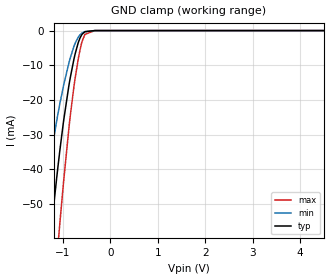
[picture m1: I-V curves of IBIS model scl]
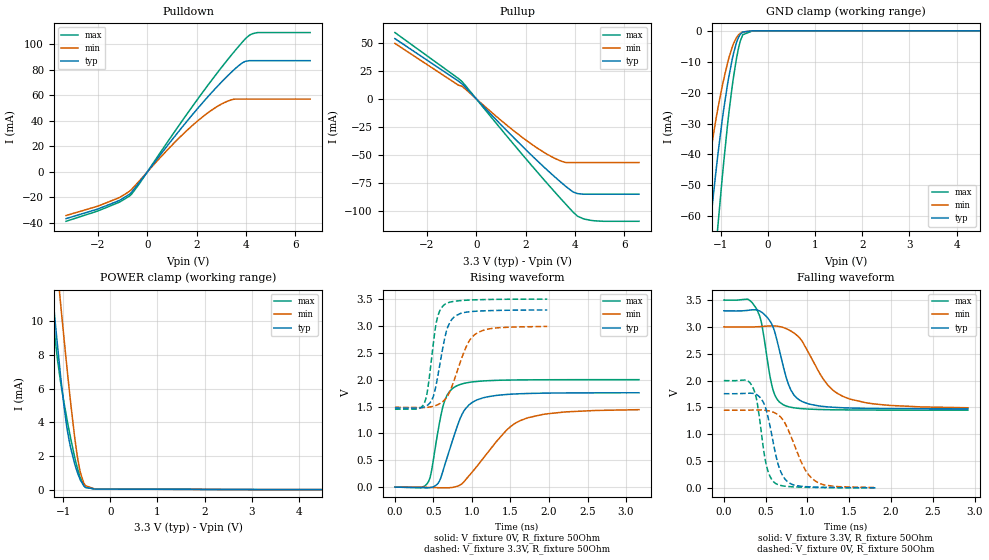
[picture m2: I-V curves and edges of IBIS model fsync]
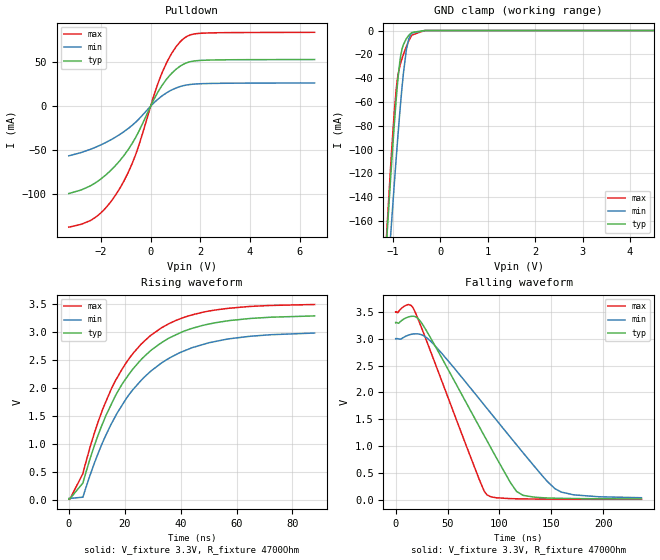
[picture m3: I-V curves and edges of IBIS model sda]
|Texas Instruments Incorporated
|50-W, 2-MHz Digital Input 4-Channel Automotive Class-D Audio Amplifier
|With Load Dump Protection and I2C Diagnostics
|Marketing part#   Digital Voltage Range   Package-type   #pins
|TPA6404   3V - 26.4V   HSSOP   56
[IBIS Ver]   4.1
[File name]   tpa6404-q1.ibs
[File Rev]   1.0
[Date]   10/27/2017
[Source]
| Texas Instruments Incorporated.
| Analog-eLab Design Center
| 12500 TI Blvd
| Dallas, TX -75243
[Notes]   Revision History:
| Rev 1.0: 9/17/2016
| - Initial version of the model
| - Model generated from simulations in SPECTRE
| - Model matched to SPICE simulation
| - C_comp although listed in numerical order of value are
|   obtained from varying PVT conditions. For PVT conditions for
|   each specific value refer the buffer description under
|   respective [Model]. IBIS model user is responsible for using
|   appropriate C_comp to simulate for Signal Integrity.
[Disclaimer]
| This model is designed as an aid for customers of Texas Instruments.
| TI and its licensors and suppliers make no warranties, either expressed
| or implied, with respect to this  model, including the warranties of
| merchantability or fitness for a particular purpose. The model is
| provided solely on an "as is" basis. The entire risk as to its quality
| and performance is with the customer.
[Copyright]
(C) Copyright 2017 Texas Instruments Incorporated.All rights reserved.
|   TPA6404_Q1DKQ
[Component]   TPA6404QDKQQ1
[Manufacturer]   TI
[Package]   |56 DKQ - HSSOP Package
|   typ   min   max
R_pkg   0.2   0.16   0.24
L_pkg   1.5nH   1.2nH   1.8nH
C_pkg   0.4pF   0.32pF   0.48pF
[Pin]  signal_name   model_name   R_pin   L_pin   C_pin
1   GND   gnd   NA   NA   NA
2   PVDD   power   NA   NA   NA
3   VBAT   power   NA   NA   NA
4   AVSS   power   NA   NA   NA
5   AVDD   power   NA   NA   NA
6   GVDD   power   NA   NA   NA
7   GVDD   power   NA   NA   NA
8   GND   gnd   NA   NA   NA
9   IN_4P   nc   NA   NA   NA
10   IN_4M   nc   NA   NA   NA
11   IN_3P   nc   NA   NA   NA
12   IN_3M   nc   NA   NA   NA
13   IN_2P   nc   NA   NA   NA
14   IN_2M   nc   NA   NA   NA
15   IN_1P   nc   NA   NA   NA
16   IN_1M   nc   NA   NA   NA
17   DVSS   gnd   NA   NA   NA
18   DVDD   power   NA   NA   NA
19   SYNC   nc   NA   NA   NA
20   SCL   scl   NA   NA   NA
21   SDA   sda   NA   NA   NA
22   I2C_ADDR0   fsync   NA   NA   NA
23   I2C_ADDR1   fsync   NA   NA   NA
24   _STANDBY   nc   NA   NA   NA
25   _MUTE   nc   NA   NA   NA
26   _FAULT   nc   NA   NA   NA
27   _WARN   nc   NA   NA   NA
28   GND   nc   NA   NA   NA
29   PVDD   power   NA   NA   NA
30   PVDD   power   NA   NA   NA
31   BST_1M   power   NA   NA   NA
32   OUT_1M   nc   NA   NA   NA
33   GND   gnd   NA   NA   NA
34   OUT_1P   nc   NA   NA   NA
35   BST_1P   power   NA   NA   NA
36   GND   gnd   NA   NA   NA
37   BST_2M   power   NA   NA   NA
38   OUT_2M   nc   NA   NA   NA
39   GND   gnd   NA   NA   NA
40   OUT_2P   nc   NA   NA   NA
41   BST_2P   power   NA   NA   NA
42   PVDD   power   NA   NA   NA
43   PVDD   power   NA   NA   NA
44   BST_3M   power   NA   NA   NA
45   OUT_3M   nc   NA   NA   NA
46   GND   gnd   NA   NA   NA
47   OUT_3P   nc   NA   NA   NA
48   BST_3P   power   NA   NA   NA
49   GND   gnd   NA   NA   NA
50   BST_4M   power   NA   NA   NA
51   OUT_4M   nc   NA   NA   NA
52   GND   gnd   NA   NA   NA
53   OUT_4P   nc   NA   NA   NA
54   BST_4P   power   NA   NA   NA
55   PVDD   power   NA   NA   NA
56   PVDD   power   NA   NA   NA
57   ThermalPad   gnd   NA   NA   NA
| Models and submodels in the file (3): scl (Input), fsync (I/O), sda (I/O_open_drain)
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|   sclk Model
[Model]   scl
Model_type   Input
Vinl = 0.99
Vinh = 2.31
|   typ   min   max
|   (nom PVT)   (fast PVT)   (slow PVT)
C_comp   6.288e-13   4.758e-13   7.537e-13
| Where nom  PVT is Nominal Process, 3.3V, 27C
|   Fast PVT is Strong Process,  3.5V, -40C
|   Slow PVT is Weak Process,   3V, 150C
[Model spec]
|subparameter
Vinl   0.99   0.90   1.05
Vinh   2.31   2.10   2.45
[Voltage Range]   3.3   3   3.5
|Junction Temperature
[Temperature Range]   27   150   -40
[Power Clamp Reference]   3.3   3   3.5
[GND Clamp Reference]   0   0   0
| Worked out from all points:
|   GND clamp passes 1 mA (typ) near -0.59 V on its own axis
[GND Clamp]
|   Voltage   I(typ)   I(min)   I(max)
-3.3V     -394.6mA   -304mA     -465.7mA
-1.544V   -99.89mA   -64.75mA   -138.1mA
-1.449V   -85.57mA   -54.72mA   -120.8mA
-1.287V   -62.45mA   -39.03mA   -92.13mA
-1.238V   -55.77mA   -34.62mA   -83.61mA
-1.105V   -39.09mA   -23.91mA   -61.71mA
-1.067V   -34.61mA   -21.1mA    -55.6mA
-877.8mV  -16.02mA   -9.452mA   -28.4mA
-769.5mV  -8.242mA   -4.556mA   -16.14mA
-642mV    -2.16mA    -1.238mA   -5.635mA
-538.5mV  -329.1uA   -291.4uA   -1.101mA
6.6V      0A         0A         0A
[POWER Clamp]
|   Voltage   I(typ)   I(min)   I(max)
-3.3V     0A         0A         0A
0V        0A         0A         0A
6.6V      0A         0A         0A
|   fsync Model
[Model]   fsync
Model_type   I/O
Polarity   Non-Inverting
Enable   Active-High
Vinl = 0.99
Vinh = 2.31
Vmeas = 1.65
Vref = 0
Cref = 2pF
Rref = 70
|   typ   min   max
|   (nom PVT)   (fast PVT)   (slow PVT)
C_comp   9.736e-13   8.094e-13   1.100e-12
| Where nom  PVT is Nominal Process, 3.3V, 27C
|   Fast PVT is Strong Process,  3.5V, -40C
|   Slow PVT is Weak Process,   3V, 150C
[Model spec]
|subparameter
Vinl   0.99   0.90   1.05
Vinh   2.31   2.10   2.45
[Voltage Range]   3.3   3   3.5
|Junction Temperature
[Temperature Range]   27   150   -40
[Pullup Reference]   3.3   3   3.5
[Pulldown Reference]   0   0   0
[Power Clamp Reference]   3.3   3   3.5
[GND Clamp Reference]   0   0   0
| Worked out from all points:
|   slope of the pulldown table from 0 to 0.495 V, typ, clamps not added: 39.4 ohm
|   slope of the pullup table from 0 to 0.495 V, typ, clamps not added: 43.1 ohm
|   GND clamp passes 1 mA (typ) near -0.58 V on its own axis
|   POWER clamp passes 1 mA (typ) near -0.70 V on its own axis
|   falling waveform, V_fixture 3.3V, R_fixture 50Ohm: 20-80 % time 195ps typ, 378ps min, 135ps max; typ from 3.3 V to 1.47 V
|   rising waveform, V_fixture 0V, R_fixture 50Ohm: 20-80 % time 257ps typ, 519ps min, 157ps max; typ from 0 V to 1.76 V
|   rising waveform, V_fixture 3.3V, R_fixture 50Ohm: 20-80 % time 149ps typ, 236ps min, 112ps max; typ from 1.47 V to 3.3 V
|   falling waveform, V_fixture 0V, R_fixture 50Ohm: 20-80 % time 154ps typ, 245ps min, 115ps max; typ from 1.76 V to 0.004 V
[Pulldown]
|   Voltage   I(typ)   I(min)   I(max)
-3.3V     -36.59mA   -34.16mA   -38.69mA
-2.079V   -29.49mA   -27.22mA   -31.04mA
-1.203V   -22.91mA   -20.65mA   -24.25mA
-647mV    -16.03mA   -13.82mA   -17.58mA
994.5mV   25.05mA    20.91mA    28.46mA
2.373V    57.15mA    45.17mA    65.81mA
2.988V    70.06mA    53mA       81.42mA
3.408V    78.14mA    56.54mA    91.58mA
3.849V    85.46mA    57.07mA    101.7mA
4.143V    87.2mA     57.07mA    107.1mA
4.481V    87.2mA     57.07mA    109.2mA
6.6V      87.2mA     57.07mA    109.2mA
[GND Clamp]
|   Voltage   I(typ)   I(min)   I(max)
-3.3V     -440mA     -341.7mA   -519.1mA
-1.534V   -111.5mA   -73.85mA   -152.9mA
-1.431V   -94.25mA   -61.6mA    -132.1mA
-1.227V   -62.33mA   -39.69mA   -92.37mA
-1.062V   -39.41mA   -24.68mA   -62.25mA
-975mV    -28.86mA   -17.95mA   -47.56mA
-867.9mV  -17.84mA   -10.78mA   -31.2mA
-762.5mV  -9.177mA   -5.256mA   -17.88mA
-633mV    -2.229mA   -1.378mA   -5.882mA
-538.5mV  -388.1uA   -364.3uA   -1.272mA
-330mV    -4.25uA    -9.019uA   -5.089uA
6.6V      0A         0A         0A
[Pullup]
|   Voltage   I(typ)   I(min)   I(max)
-3.3V     53.6mA     49.34mA    59.01mA
-724mV    15.74mA    12.1mA     18.05mA
-588mV    13.44mA    11.21mA    15.53mA
1.284V    -29.46mA   -24.34mA   -34.44mA
2.553V    -56.88mA   -45.07mA   -67.28mA
2.973V    -65.43mA   -50.65mA   -77.83mA
3.51V     -75.83mA   -56.07mA   -91.03mA
3.901V    -82.68mA   -56.8mA    -100.4mA
4.095V    -84.42mA   -56.8mA    -104.4mA
4.353V    -85.03mA   -56.8mA    -107mA
4.795V    -85.03mA   -56.8mA    -108.7mA
6.6V      -85.03mA   -56.8mA    -109.2mA
[POWER Clamp]
|   Voltage   I(typ)   I(min)   I(max)
-3.3V     78.62mA    81.34mA    82.98mA
-1.294V   13.67mA    18.15mA    12.46mA
-1.224V   11.54mA    16.02mA    10.33mA
-1.123V   8.586mA    13.02mA    7.731mA
-1.056V   6.746mA    11.05mA    6.397mA
-976.8mV  4.8mA      8.789mA    5.06mA
-871mV    2.867mA    5.898mA    3.45mA
-696mV    993.8uA    1.895mA    1.238mA
-636.5mV  569.5uA    1.011mA    691.4uA
-525mV    128.3uA    227.9uA    131.5uA
-264mV    32.56uA    34.05uA    33.82uA
6.6V      0A         0A         0A
[Ramp]
R_load = 50
|   typ   min   max
dV/dt_r   1.05398/2.56961e-10   0.869396/5.22864e-10   1.20008/1.57028e-10
dV/dt_f   1.09538/1.94389e-10   0.908068/3.80996e-10   1.2297/1.34491e-10
[Falling Waveform]
V_fixture = 3.3V
V_fixture_min = 3V
V_fixture_max = 3.5V
R_fixture = 50Ohm
|   Time   V(typ)   V(min)   V(max)
0s        3.3V       3V         3.5V
281.6ps   3.308V     2.998V     3.519V
382.7ps   3.32V      3.002V     3.358V
452.5ps   3.275V     3.009V     3.06V
590ps     2.996V     3.02V      1.822V
729.9ps   2.15V      2.979V     1.537V
909.1ps   1.634V     2.791V     1.481V
1.197ns   1.517V     2.013V     1.46V
1.428ns   1.494V     1.704V     1.455V
2.92ns    1.474V     1.494V     1.45V
[Rising Waveform]
V_fixture = 0V
V_fixture_min = 0V
V_fixture_max = 0V
R_fixture = 50Ohm
|   Time   V(typ)   V(min)   V(max)
0s        345.2pV    23.28nV    146.2pV
432.7ps   -12.69mV   -4.635mV   96.19mV
471.2ps   -5.458mV   -6.65mV    271.6mV
564.5ps   79.77mV    -11.33mV   1.087V
644.3ps   400.1mV    -13.85mV   1.602V
816.8ps   1.164V     20.23mV    1.894V
919.8ps   1.465V     140.5mV    1.938V
1.062ns   1.621V     383.8mV    1.966V
1.635ns   1.738V     1.242V     1.995V
3.168ns   1.756V     1.441V     2V
[Rising Waveform]
V_fixture = 3.3V
V_fixture_min = 3V
V_fixture_max = 3.5V
R_fixture = 50Ohm
|   Time   V(typ)   V(min)   V(max)
0s        1.474V     1.486V     1.45V
382.7ps   1.495V     1.481V     1.569V
429ps     1.531V     1.487V     1.856V
496.4ps   1.679V     1.504V     2.646V
540ps     1.94V      1.524V     3.083V
647.9ps   2.784V     1.629V     3.401V
771.7ps   3.171V     2.003V     3.458V
911.6ps   3.253V     2.567V     3.477V
1.039ns   3.272V     2.841V     3.485V
1.977ns   3.297V     2.991V     3.498V
[Falling Waveform]
V_fixture = 0V
V_fixture_min = 0V
V_fixture_max = 0V
R_fixture = 50Ohm
|   Time   V(typ)   V(min)   V(max)
0s        1.757V     1.449V     2V
346ps     1.763V     1.452V     1.876V
399.8ps   1.733V     1.454V     1.584V
510ps     1.438V     1.445V     416.5mV
616.5ps   649mV      1.394V     86.83mV
681.2ps   303.6mV    1.319V     46.63mV
765.1ps   113mV      1.1V       27.92mV
972.2ps   25.29mV    342mV      13.23mV
1.087ns   16.68mV    137mV      9.613mV
1.817ns   3.697mV    8.046mV    2.24mV
|   sda Model
[Model]   sda
Model_type   I/O_open_drain
Polarity   Non-Inverting
Vinl = 0.99
Vinh = 2.31
Vmeas = 1.65
Vref = 3.3
Cref = 2pF
Rref = 4700
|   typ   min   max
|   (nom PVT)   (fast PVT)   (slow PVT)
C_comp   1.956e-12   1.803e-12   2.012e-12
| Where nom  PVT is Nominal Process, 3.3V, 27C
|   Fast PVT is Strong Process,  3.5V, -40C
|   Slow PVT is Weak Process,   3V, 150C
[Model spec]
|subparameter
Vinl   0.99   0.90   1.05
Vinh   2.31   2.10   2.45
[Voltage Range]   3.3   3   3.5
|Junction Temperature
[Temperature Range]   27   150   -40
[Pullup Reference]   3.3   3   3.5
[Pulldown Reference]   0   0   0
[Power Clamp Reference]   3.3   3   3.5
[GND Clamp Reference]   0   0   0
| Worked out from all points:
|   slope of the pulldown table from 0 to 0.495 V, typ, clamps not added: 19.9 ohm
|   falling waveform, V_fixture 3.3V, R_fixture 4700Ohm: 20-80 % time 55.9ns typ, 75ns min, 41.1ns max; typ from 3.3 V to 0.016 V
|   rising waveform, V_fixture 3.3V, R_fixture 4700Ohm: 20-80 % time 21.3ns typ, 22.8ns min, 19.9ns max; typ from 0.012 V to 3.29 V
[Pulldown]
|   Voltage   I(typ)   I(min)   I(max)
-3.3V     -99.17mA   -56.36mA   -137.3mA
-2.187V   -86.26mA   -46.17mA   -125.4mA
-1.653V   -74.09mA   -38.9mA    -110.1mA
-1.267V   -62.56mA   -32.47mA   -94.28mA
-914.1mV  -49.53mA   -25.48mA   -75.62mA
-615mV    -35.89mA   -18.39mA   -55.51mA
141mV     8.345mA    4.125mA    13.44mA
462.5mV   23.86mA    11.81mA    38.32mA
858mV     37.74mA    18.62mA    60.61mA
1.341V    47.93mA    23.46mA    77.07mA
2.041V    52.03mA    25.53mA    82.82mA
6.6V      52.99mA    26.37mA    83.85mA
[GND Clamp]
|   Voltage   I(typ)   I(min)   I(max)
-3.3V     -1.775A    -1.719A    -1.841A
-1.13V    -175.7mA   -220.7mA   -169.6mA
-1.056V   -129mA     -177.2mA   -119.8mA
-1.026V   -111mA     -160.1mA   -100.8mA
-927mV    -56.11mA   -105.5mA   -48.12mA
-851.4mV  -25.44mA   -67.54mA   -29.68mA
-780mV    -11.99mA   -36.69mA   -20.21mA
-717mV    -6.878mA   -16.61mA   -13.39mA
-666mV    -4.086mA   -7.158mA   -8.704mA
-594.5mV  -1.595mA   -2.044mA   -3.733mA
-330mV    -7.451uA   -31.37uA   -5.074uA
6.6V      0A         0A         0A
[POWER Clamp]
|   Voltage   I(typ)   I(min)   I(max)
-3.3V     0A         0A         0A
0V        0A         0A         0A
6.6V      0A         0A         0A
[Ramp]
R_load = 4700
|   typ   min   max
dV/dt_r   1.97304/2.15244e-08   1.78711/2.31201e-08   2.09541/1.99936e-08
dV/dt_f   1.97191/5.58691e-08   1.78233/7.52238e-08   2.09515/4.1067e-08
[Falling Waveform]
V_fixture = 3.3V
V_fixture_min = 3V
V_fixture_max = 3.5V
R_fixture = 4700Ohm
|   Time   V(typ)   V(min)   V(max)
0s        3.3V       3V         3.5V
12.24ns   3.404V     3.065V     3.636V
17.68ns   3.416V     3.088V     3.538V
36.09ns   2.93V      2.905V     2.638V
80ns      1.381V     1.892V     404.2mV
87.93ns   1.102V     1.702V     92.68mV
110.5ns   321.6mV    1.165V     21.71mV
122.5ns   84.68mV    881.6mV    16.77mV
159.5ns   27.16mV    144.9mV    11.35mV
236.8ns   15.65mV    38.4mV     8.697mV
[Rising Waveform]
V_fixture = 3.3V
V_fixture_min = 3V
V_fixture_max = 3.5V
R_fixture = 4700Ohm
|   Time   V(typ)   V(min)   V(max)
0s        11.52mV    21.15mV    7.585mV
5.031ns   296.6mV    44.48mV    465.6mV
10.49ns   1.156V     828.4mV    1.393V
15.83ns   1.771V     1.413V     2.046V
21.79ns   2.263V     1.895V     2.539V
29.02ns   2.655V     2.285V     2.927V
38.48ns   2.953V     2.599V     3.21V
50.02ns   3.141V     2.806V     3.374V
65.06ns   3.243V     2.924V     3.458V
87.93ns   3.288V     2.981V     3.492V
